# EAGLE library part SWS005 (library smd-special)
SMD Dip Switch 5 pol.
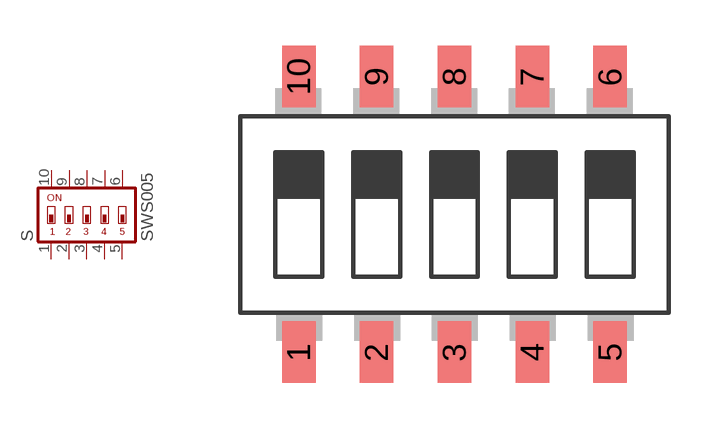
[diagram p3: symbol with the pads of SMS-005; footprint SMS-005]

Designator prefix S

## SWS005  [SMS-005]
1  1  pas
2  2  pas
3  3  pas
4  4  pas
5  5  pas
6  6  pas
7  7  pas
8  8  pas
9  9  pas
10  10  pas

## Footprint SMS-005 (pad centres in mm)
DIP SWITCH
smd 1.092 x 2.007: 1 -5.08,-4.496; 2 -2.54,-4.496; 3 0,-4.496; 4 2.54,-4.496; 5 5.08,-4.496; 6 5.08,4.496; 7 2.54,4.496; 8 0,4.496; 9 -2.54,4.496; 10 -5.08,4.496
